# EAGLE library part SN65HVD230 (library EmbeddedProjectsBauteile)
CAN Transceiver
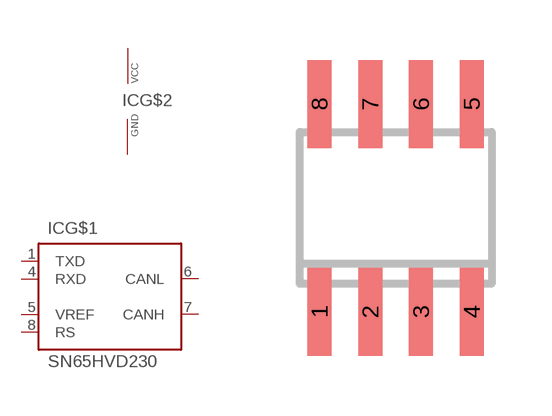
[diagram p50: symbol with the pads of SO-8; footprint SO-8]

Designator prefix IC; gates G$1=SN65HVD G$2=VCC-GND

## SN65HVD230D  [SO-8]
1  G$1:TXD
2  G$2:GND  pwr
3  G$2:+5V  pwr
4  G$1:RXD
5  G$1:VREF
6  G$1:CANL
7  G$1:CANH
8  G$1:RS

## Footprint SO-8 (pad centres in mm)
smd 0.6 x 2.2: 1 -1.905,-2.6; 2 -0.635,-2.6; 3 0.635,-2.6; 4 1.905,-2.6; 5 1.905,2.6; 6 0.635,2.6; 7 -0.635,2.6; 8 -1.905,2.6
